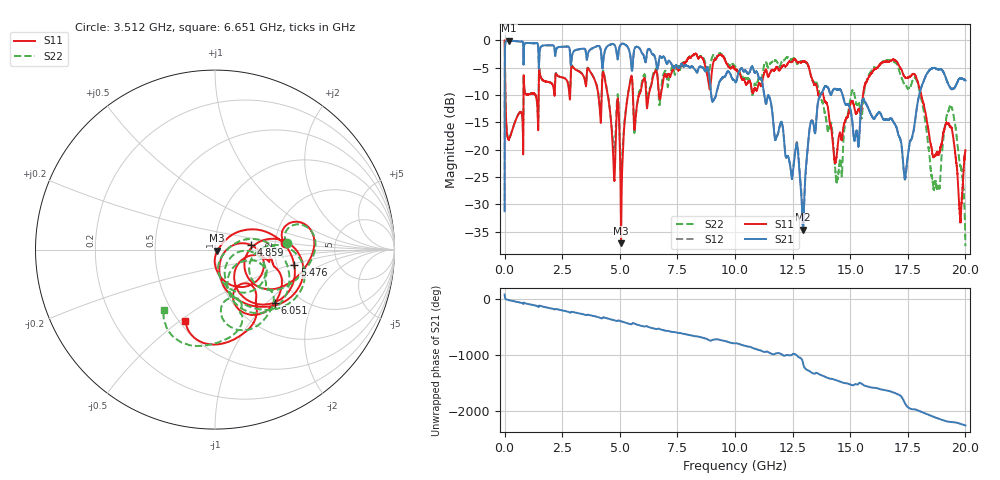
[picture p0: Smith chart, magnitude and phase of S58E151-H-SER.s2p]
!{S58E151}
!Johanson Technology Inc.
!www.johansontechnology.com
!Test Board Conditions:
!Substrate Type  RO4350B
!Substrate Thickness  60 mil
!Substrate Dk  3.66
!TL Type: GCPW
!TL Trace Width  115 mil
!TL Gap  52 mil
!Electrode orientation  Horizontal
!DUT TOPOLOGY	SERIES
!Mounting Pad LxW  55x428 mil
! Created Wed Apr 14 11:13:49 2021
# mhz S ma R 50
! 2 Port Network Data from SP1.SP block
! freq  magS11  angS11  magS21  angS21  magS12  angS12  magS22  angS22
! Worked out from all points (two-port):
!   20001 points, 300 kHz to 20 GHz, reference 50 ohm
!   highest |S21| = -0.08 dB at 202.3 MHz (marker M1); lowest = -34.7 dB at 12.96 GHz (marker M2)
!   |S21| within 3 dB of the highest: 10.86 MHz to 818.9 MHz (808 MHz wide, 195 % of centre); 1.506 GHz to 2.85 GHz (1.344 GHz wide, 61.7 % of centre)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
!   lowest |S11| = -37.1 dB at 5.055 GHz (marker M3), VSWR 1.03, Z = 51.3 - j0.574 ohm
!   |S11| at or under -10 dB: 4.477 GHz to 5.352 GHz (874.4 MHz wide, 17.8 % of centre); 13.83 GHz to 15.55 GHz (1.725 GHz wide, 11.7 % of centre); 18.08 GHz to end of sweep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
!   |S22| runs from -37.7 to -0.1 dB; largest |S21 - S12| = 0.0086
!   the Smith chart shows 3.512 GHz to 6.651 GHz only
!   S11 on the Smith chart (normalised r, x): 3.512 GHz: 2.28, +0.20; 4.859 GHz: 1.50, +0.08; 5.476 GHz: 2.50, -0.55; 6.051 GHz: 1.50, -1.11; 6.651 GHz: 0.54, -0.52
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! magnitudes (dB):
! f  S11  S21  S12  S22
! 300 kHz  0.0  -31.3  -31.2  -0.1
! 202.3 MHz  -17.9  -0.1  -0.1  -17.9
! 3.334 GHz  -6.0  -1.6  -1.6  -6.0
! 3.512 GHz  -8.1  -1.9  -1.9  -7.9
! 4.859 GHz  -13.9  -2.2  -2.2  -12.6
! 5.055 GHz  -37.1  -0.7  -0.7  -25.4
! 5.476 GHz  -6.9  -3.5  -3.5  -7.0
! 6.051 GHz  -7.0  -3.0  -3.0  -6.3
! 6.651 GHz  -7.4  -5.2  -5.1  -7.2
! 6.667 GHz  -8.2  -4.7  -4.7  -8.4
! 10 GHz  -5.3  -7.6  -7.6  -4.8
! 11.08 GHz  -8.0  -7.1  -7.1  -7.0
! 12.96 GHz  -3.9  -34.7  -34.2  -3.9
! 13.33 GHz  -6.9  -14.7  -14.6  -7.1
! 14.43 GHz  -20.4  -9.0  -9.0  -25.7
! 15.07 GHz  -11.2  -14.1  -14.2  -9.4
! 16.67 GHz  -4.0  -14.6  -14.5  -3.6
! 17.39 GHz  -6.9  -25.1  -25.3  -8.2
! 18.69 GHz  -21.1  -5.1  -5.1  -25.8
! 19.4 GHz  -16.0  -8.9  -8.9  -12.3
! 19.77 GHz  -32.8  -7.0  -6.9  -23.0
! 20 GHz  -20.1  -7.4  -7.3  -37.7
